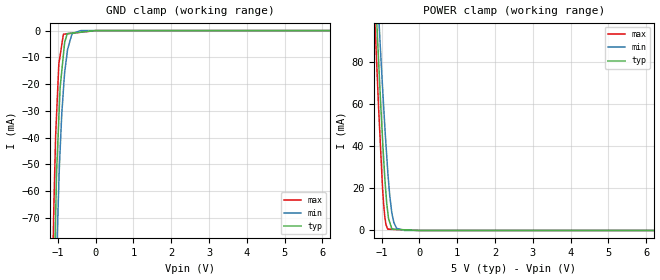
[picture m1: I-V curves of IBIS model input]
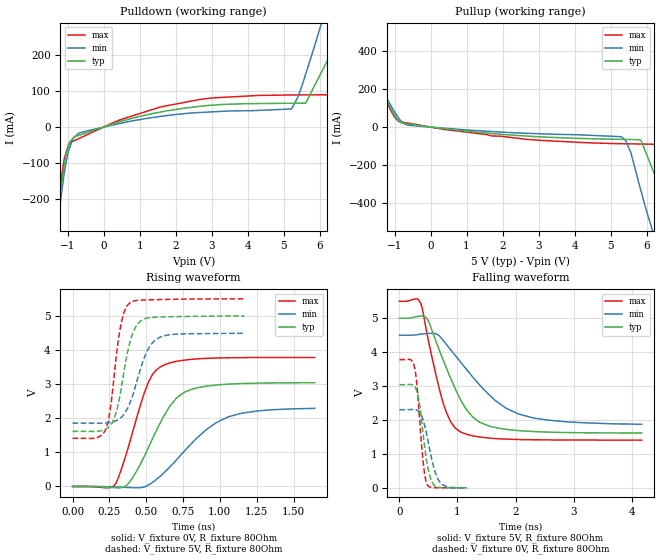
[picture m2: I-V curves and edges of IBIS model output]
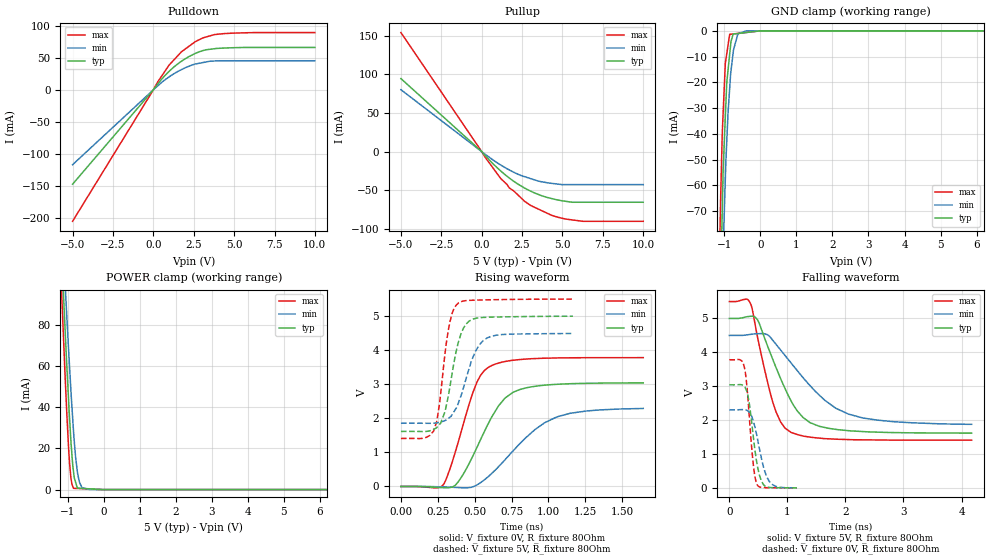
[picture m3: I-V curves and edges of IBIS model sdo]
|Texas Instruments Incorporated
| Precision Low-Side, Digital Current Sensor and Voltage Monitor
| Marketing part#   Digital Voltage Range   Package-type   #pins
| LMP92064   4.5V-5.5V   LLP   16
[IBIS Ver]   4.1
[File name]   lmp92064.ibs
[File Rev]   1.0
[Date]   5/30/2013
[Source]
| Texas Instruments Incorporated.
| Analog-eLab Design Center, HPA
| 12500 TI Blvd
| Dallas, TX -75243
[Notes]   Revision History:
| Rev 1.0: 5/30/2013
| - Initial version of the model
| - Model generated from simulations in SPECTRE
| - Model matched to SPICE simulation
| - C_comp although listed in numerical order of value are
|   obtained from varying PVT conditions. For PVT conditions for
|   each specific value refer the buffer description under
|   respective [Model]. IBIS model user is responsible for using
|   appropriate C_comp to simulate for Signal Integrity.
| - Model names contains the model for 5V [4.5V and 5.5V].
[Disclaimer]
| This model is designed as an aid for customers of Texas Instruments.
| TI and its licensors and suppliers make no warranties, either expressed
| or implied, with respect to this  model, including the warranties of
| merchantability or fitness for a particular purpose. The model is
| provided solely on an "as is" basis. The entire risk as to its quality
| and performance is with the customer.
[Copyright]
(C) Copyright 2013 Texas Instruments Incorporated.All rights reserved.
|   LMP92064LLP
[Component]   LMP92064LLP
[Manufacturer]   TI
[Package]   |16 LLP  package
|   typ   min   max
R_pkg   0.01   0.008   0.12
L_pkg   1.0nH   0.8nH   1.2nH
C_pkg   0.2pF   0.16pF   0.24pF
[Pin]  signal_name   model_name   R_pin   L_pin   C_pin
1   REFC   nc   NA   NA   NA
2   REFG   gnd   NA   NA   NA
3   INCP   nc   NA   NA   NA
4   INCN   nc   NA   NA   NA
5   INVP   nc   NA   NA   NA
6   INVG   gnd   NA   NA   NA
7   GND   gnd   NA   NA   NA
8   VDD   power   NA   NA   NA
9   VDIG   power   NA   NA   NA
10   DGND   gnd   NA   NA   NA
11   SDO   sdo   NA   NA   NA
12   SDI   input   NA   NA   NA
13   SCLK   input   NA   NA   NA
14   CSB   input   NA   NA   NA
15   Reserved   output   NA   NA   NA
16   RESET   input   NA   NA   NA
1000   DAP   nc   NA   NA   NA
| Models and submodels in the file (3): input (Input), output (Output), sdo (3-state)
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|   input Model
[Model]   input
Model_type   Input
Vinl = 0.8
Vinh = 2
|   typ   min   max
|   (nom PVT)   (fast PVT)   (slow PVT)
C_comp   6.249e-13   6.001e-13   6.512e-13
| Where nom  PVT is Nominal Process, 5V, 27C
|   Fast PVT is Strong Process,  5.5V, -40C
|   Slow PVT is Weak Process,   4.5V, 105C
[Voltage Range]   5   4.5   5.5
|Junction Temperature
[Temperature Range]   27   105   -40
[Power Clamp Reference]   5   4.5   5.5
[GND Clamp Reference]   0   0   0
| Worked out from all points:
|   GND clamp passes 1 mA (typ) near -0.67 V on its own axis
|   POWER clamp passes 1 mA (typ) near -0.73 V on its own axis
[GND Clamp]
|   Voltage   I(typ)   I(min)   I(max)
-5V       -2.28A     -2.11A     -2.479A
-1.145V   -123.7mA   -156.3mA   -94.06mA
-1.106V   -99.37mA   -129.1mA   -66.13mA
-1.062V   -71.6mA    -101.5mA   -41.27mA
-1.03V    -52.11mA   -83.03mA   -30.4mA
-974mV    -32.98mA   -57.5mA    -12.58mA
-940mV    -21.36mA   -44.82mA   -9.427mA
-853mV    -9.052mA   -22.29mA   -1.371mA
-743mV    -1.114mA   -7.12mA    -1.194mA
-639.5mV  -959.2uA   -1.856mA   -1.027mA
-392mV    -588uA     -4.464uA   -629.5uA
10V       0A         0A         0A
[POWER Clamp]
|   Voltage   I(typ)   I(min)   I(max)
-5V       1.561A     1.48A      1.644A
-1.247V   144.2mA    160.8mA    129.1mA
-1.079V   80.59mA    102.8mA    58.18mA
-1.036V   64.35mA    87.98mA    42.43mA
-979.5mV  45.09mA    69.76mA    21.91mA
-946.5mV  34.55mA    59.5mA     12.74mA
-908mV    23.21mA    47.59mA    5.515mA
-836.5mV  8.707mA    28.01mA    619.8uA
-783.5mV  3.839mA    16.46mA    580.5uA
-675.5mV  574.4uA    3.786mA    500.4uA
-392mV    333.3uA    0A         290.3uA
10V       0A         0A         0A
|   output Model
[Model]   output
Model_type   Output
Polarity   Non-Inverting
Vmeas = 2.5
Vref = 0
Cref = 2pF
Rref = 95
|   typ   min   max
|   (nom PVT)   (fast PVT)   (slow PVT)
C_comp   3.855e-13   3.827e-13   3.962e-13
| Where nom  PVT is Nominal Process, 5V, 27C
|   Fast PVT is Strong Process,  5.5V, -40C
|   Slow PVT is Weak Process,   4.5V, 105C
[Voltage Range]   5   4.5   5.5
|Junction Temperature
[Temperature Range]   27   105   -40
[Pullup Reference]   5   4.5   5.5
[Pulldown Reference]   0   0   0
[Power Clamp Reference]   5   4.5   5.5
[GND Clamp Reference]   0   0   0
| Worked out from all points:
|   slope of the pulldown table from 0 to 0.75 V, typ, clamps not added: 32.6 ohm
|   slope of the pullup table from 0 to 0.75 V, typ, clamps not added: 45 ohm
|   falling waveform, V_fixture 5V, R_fixture 80Ohm: 20-80 % time 533ps typ, 865ps min, 349ps max; typ from 5 V to 1.62 V
|   rising waveform, V_fixture 0V, R_fixture 80Ohm: 20-80 % time 220ps typ, 328ps min, 162ps max; typ from 0 V to 3.04 V
|   rising waveform, V_fixture 5V, R_fixture 80Ohm: 20-80 % time 92ps typ, 121ps min, 71.1ps max; typ from 1.62 V to 5 V
|   falling waveform, V_fixture 0V, R_fixture 80Ohm: 20-80 % time 138ps typ, 182ps min, 108ps max; typ from 3.04 V to 0.004 V
[Pulldown]
|   Voltage   I(typ)   I(min)   I(max)
-5V       -2.28A     -2.11A     -2.479A
-1.508V   -435.2mA   -429.7mA   -450.3mA
-1.25V    -223.8mA   -242.2mA   -212.1mA
-963mV    -49.14mA   -62.51mA   -44.37mA
-702.5mV  -23.2mA    -17.33mA   -32.32mA
1.578V    41.51mA    29.56mA    55.6mA
5.215V    65.86mA    50.03mA    88.71mA
5.61V     66.03mA    146.1mA    88.99mA
6.034V    148.7mA    282mA      89.21mA
6.457V    266.3mA    425.7mA    101.7mA
6.764V    379.2mA    532.7mA    202.9mA
10V       1.567A     1.659A     1.455A
[Pullup]
|   Voltage   I(typ)   I(min)   I(max)
-5V       1.561A     1.48A      1.644A
-1.25V    149.8mA    163.4mA    142.7mA
-891.5mV  34.32mA    49mA       30.06mA
-644mV    17.3mA     11.18mA    21.66mA
5.301V    -64.75mA   -50.94mA   -87.7mA
5.561V    -65.55mA   -133.1mA   -88.48mA
5.845V    -69.13mA   -336.3mA   -89.34mA
6.245V    -260.4mA   -594.7mA   -90.55mA
6.594V    -527.1mA   -787.1mA   -140mA
6.979V    -778.6mA   -998.5mA   -459.6mA
7.194V    -896.3mA   -1.102A    -639.2mA
10V       -2.286A    -2.31A     -2.248A
[Ramp]
R_load = 80
|   typ   min   max
dV/dt_r   1.82542/2.2047e-10   1.38355/3.31567e-10   2.26924/1.61805e-10
dV/dt_f   2.03065/5.33123e-10   1.58605/8.72476e-10   2.45372/3.48746e-10
[Falling Waveform]
V_fixture = 5V
V_fixture_min = 4.5V
V_fixture_max = 5.5V
R_fixture = 80Ohm
|   Time   V(typ)   V(min)   V(max)
0s        5V         4.5V       5.5V
359.5ps   5.063V     4.529V     5.46V
488.6ps   4.955V     4.549V     4.429V
750.6ps   3.784V     4.353V     2.517V
883.4ps   3.227V     4.071V     1.949V
1.066ns   2.562V     3.683V     1.636V
1.387ns   1.929V     3.025V     1.5V
2.055ns   1.689V     2.177V     1.427V
2.846ns   1.633V     1.952V     1.412V
4.174ns   1.617V     1.877V     1.41V
[Rising Waveform]
V_fixture = 0V
V_fixture_min = 0V
V_fixture_max = 0V
R_fixture = 80Ohm
|   Time   V(typ)   V(min)   V(max)
0s        985.4pV    2.368nV    893.5pV
293.7ps   -38.36mV   -14.21mV   89.78mV
385.9ps   122.2mV    -31.8mV    1.264V
516.1ps   1.152V     47.38mV    3.068V
605.8ps   1.957V     341.5mV    3.528V
661.5ps   2.363V     577.9mV    3.622V
761.4ps   2.769V     1.048V     3.705V
910.4ps   2.941V     1.674V     3.755V
1.058ns   2.999V     2.043V     3.773V
1.644ns   3.04V      2.29V      3.782V
[Rising Waveform]
V_fixture = 5V
V_fixture_min = 4.5V
V_fixture_max = 5.5V
R_fixture = 80Ohm
|   Time   V(typ)   V(min)   V(max)
0s        1.616V     1.857V     1.41V
220.9ps   1.673V     1.857V     1.625V
261.9ps   1.822V     1.882V     2.432V
307.2ps   2.361V     1.954V     4.191V
331.9ps   2.921V     2.031V     4.825V
392.1ps   4.268V     2.479V     5.393V
442.7ps   4.772V     3.176V     5.456V
503.6ps   4.93V      3.953V     5.469V
585.2ps   4.967V     4.362V     5.478V
1.167ns   4.998V     4.491V     5.499V
[Falling Waveform]
V_fixture = 0V
V_fixture_min = 0V
V_fixture_max = 0V
R_fixture = 80Ohm
|   Time   V(typ)   V(min)   V(max)
0s        3.042V     2.306V     3.782V
198.1ps   3.048V     2.31V      3.771V
261.9ps   2.989V     2.31V      3.546V
293.7ps   2.884V     2.297V     3.163V
322.9ps   2.703V     2.268V     2.593V
414.8ps   1.496V     1.972V     662.1mV
487.8ps   609.6mV    1.426V     68.3mV
583.6ps   107.4mV    654.1mV    10.78mV
689.7ps   15.73mV    189.5mV    6.238mV
1.163ns   3.524mV    4.697mV    2.607mV
|   sdo Model
[Model]   sdo
Model_type   3-state
Polarity   Non-Inverting
Vmeas = 2.5
Vref = 0
Cref = 20pF
Rref = 95
|   typ   min   max
|   (nom PVT)   (fast PVT)   (slow PVT)
C_comp   4.605e-13   4.436e-13   4.946e-13
| Where nom  PVT is Nominal Process, 5V, 27C
|   Fast PVT is Strong Process,  5.5V, -40C
|   Slow PVT is Weak Process,   4.5V, 105C
[Voltage Range]   5   4.5   5.5
|Junction Temperature
[Temperature Range]   27   105   -40
[Pullup Reference]   5   4.5   5.5
[Pulldown Reference]   0   0   0
[Power Clamp Reference]   5   4.5   5.5
[GND Clamp Reference]   0   0   0
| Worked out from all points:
|   slope of the pulldown table from 0 to 0.75 V, typ, clamps not added: 32.5 ohm
|   slope of the pullup table from 0 to 0.75 V, typ, clamps not added: 44.7 ohm
|   GND clamp passes 1 mA (typ) near -0.60 V on its own axis
|   POWER clamp passes 1 mA (typ) near -0.74 V on its own axis
|   falling waveform, V_fixture 5V, R_fixture 80Ohm: 20-80 % time 533ps typ, 865ps min, 349ps max; typ from 5 V to 1.62 V
|   rising waveform, V_fixture 0V, R_fixture 80Ohm: 20-80 % time 220ps typ, 328ps min, 162ps max; typ from 0 V to 3.04 V
|   rising waveform, V_fixture 5V, R_fixture 80Ohm: 20-80 % time 92ps typ, 121ps min, 71.1ps max; typ from 1.62 V to 5 V
|   falling waveform, V_fixture 0V, R_fixture 80Ohm: 20-80 % time 138ps typ, 182ps min, 108ps max; typ from 3.04 V to 0.004 V
[Pulldown]
|   Voltage   I(typ)   I(min)   I(max)
-5V       -146.9mA   -116.6mA   -204.8mA
0V        0A         0A         0A
258mV     8.765mA    5.876mA    11.8mA
978.5mV   28.87mA    20.25mA    38.73mA
1.738V    44.54mA    31.51mA    59.27mA
2.645V    57.3mA     40.49mA    75.74mA
3.068V    61.19mA    42.54mA    81.01mA
3.795V    64.16mA    45mA       86.16mA
6.258V    66.07mA    45.35mA    89.27mA
10V       66.07mA    45.35mA    89.27mA
[GND Clamp]
|   Voltage   I(typ)   I(min)   I(max)
-5V       -2.28A     -2.11A     -2.479A
-1.145V   -123.7mA   -156.2mA   -94.06mA
-1.106V   -99.37mA   -129.3mA   -66.13mA
-1.062V   -71.53mA   -101.4mA   -41.26mA
-1.026V   -51.04mA   -81.13mA   -29.29mA
-974mV    -33.34mA   -57.43mA   -12.57mA
-935mV    -20.2mA    -43.17mA   -8.962mA
-853mV    -9.02mA    -22.24mA   -1.368mA
-747.5mV  -1.246mA   -7.467mA   -1.199mA
-639.5mV  -1.066mA   -1.847mA   -1.025mA
-392mV    -653.3uA   0A         -628.2uA
10V       0A         0A         0A
[Pullup]
|   Voltage   I(typ)   I(min)   I(max)
-5V       94.53mA    80.16mA    154.2mA
0V        0A         0A         0A
1.171V    -25mA      -17.33mA   -34.73mA
1.56V     -31.86mA   -22.15mA   -42.51mA
1.718V    -34.41mA   -23.88mA   -47.28mA
1.993V    -38.62mA   -26.89mA   -51.17mA
2.645V    -47.18mA   -32.45mA   -64.21mA
3.28V     -53.7mA    -36.72mA   -72.26mA
4.339V    -60.9mA    -41.19mA   -82.66mA
5.186V    -64.4mA    -42.81mA   -87.37mA
6.253V    -65.64mA   -42.81mA   -90.32mA
10V       -65.64mA   -42.81mA   -90.32mA
[POWER Clamp]
|   Voltage   I(typ)   I(min)   I(max)
-5V       1.561A     1.48A      1.644A
-1.247V   144.2mA    160.8mA    129.1mA
-1.079V   80.59mA    102.8mA    58.18mA
-1.036V   64.36mA    88mA       41.57mA
-946.5mV  34.52mA    59.51mA    12.74mA
-908mV    23.14mA    47.61mA    5.512mA
-836.5mV  8.603mA    28.11mA    623.2uA
-779mV    3.539mA    15.66mA    580.3uA
-725mV    705.3uA    7.916mA    540.1uA
-671mV    652.7uA    3.555mA    499.8uA
-392mV    381.3uA    0A         291.8uA
10V       0A         0A         0A
[Ramp]
R_load = 80
|   typ   min   max
dV/dt_r   1.82542/2.2047e-10   1.38355/3.31567e-10   2.26924/1.61805e-10
dV/dt_f   2.03065/5.33123e-10   1.58605/8.72476e-10   2.45372/3.48746e-10
[Falling Waveform]
V_fixture = 5V
V_fixture_min = 4.5V
V_fixture_max = 5.5V
R_fixture = 80Ohm
|   Time   V(typ)   V(min)   V(max)
0s        5V         4.5V       5.5V
359.5ps   5.063V     4.529V     5.46V
488.6ps   4.955V     4.549V     4.429V
750.6ps   3.784V     4.353V     2.517V
883.4ps   3.227V     4.071V     1.949V
1.066ns   2.562V     3.683V     1.636V
1.387ns   1.929V     3.025V     1.5V
2.055ns   1.689V     2.177V     1.427V
2.846ns   1.633V     1.952V     1.412V
4.174ns   1.617V     1.877V     1.41V
[Rising Waveform]
V_fixture = 0V
V_fixture_min = 0V
V_fixture_max = 0V
R_fixture = 80Ohm
|   Time   V(typ)   V(min)   V(max)
0s        985.4pV    2.368nV    893.5pV
293.7ps   -38.36mV   -14.21mV   89.78mV
385.9ps   122.2mV    -31.8mV    1.264V
516.1ps   1.152V     47.38mV    3.068V
605.8ps   1.957V     341.5mV    3.528V
661.5ps   2.363V     577.9mV    3.622V
761.4ps   2.769V     1.048V     3.705V
910.4ps   2.941V     1.674V     3.755V
1.058ns   2.999V     2.043V     3.773V
1.644ns   3.04V      2.29V      3.782V
[Rising Waveform]
V_fixture = 5V
V_fixture_min = 4.5V
V_fixture_max = 5.5V
R_fixture = 80Ohm
|   Time   V(typ)   V(min)   V(max)
0s        1.616V     1.857V     1.41V
220.9ps   1.673V     1.857V     1.625V
261.9ps   1.822V     1.882V     2.432V
307.2ps   2.361V     1.954V     4.191V
331.9ps   2.921V     2.031V     4.825V
392.1ps   4.268V     2.479V     5.393V
442.7ps   4.772V     3.176V     5.456V
503.6ps   4.93V      3.953V     5.469V
585.2ps   4.967V     4.362V     5.478V
1.167ns   4.998V     4.491V     5.499V
[Falling Waveform]
V_fixture = 0V
V_fixture_min = 0V
V_fixture_max = 0V
R_fixture = 80Ohm
|   Time   V(typ)   V(min)   V(max)
0s        3.042V     2.306V     3.782V
198.1ps   3.048V     2.31V      3.771V
261.9ps   2.989V     2.31V      3.546V
293.7ps   2.884V     2.297V     3.163V
322.9ps   2.703V     2.268V     2.593V
414.8ps   1.496V     1.972V     662.1mV
487.8ps   609.6mV    1.426V     68.3mV
583.6ps   107.4mV    654.1mV    10.78mV
689.7ps   15.73mV    189.5mV    6.238mV
1.163ns   3.524mV    4.697mV    2.507mV
